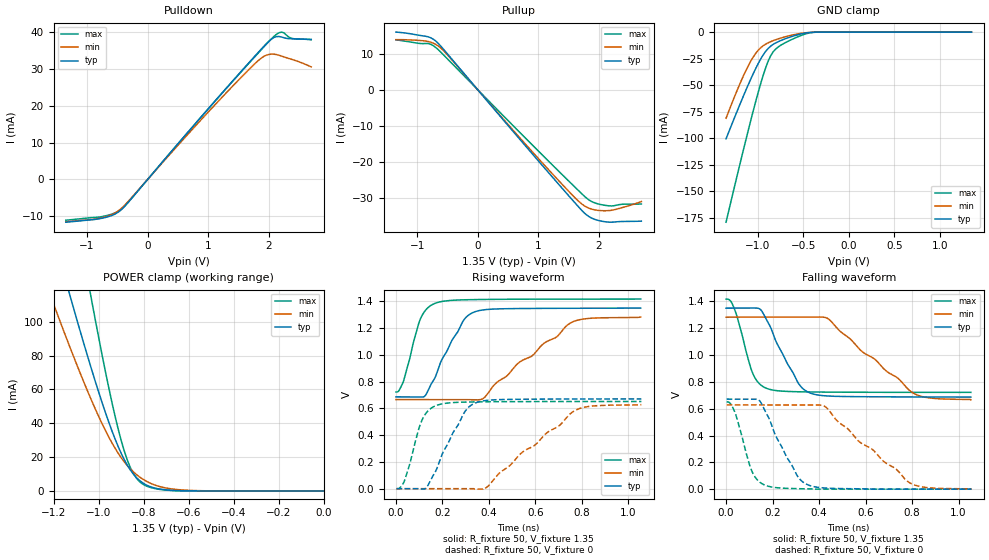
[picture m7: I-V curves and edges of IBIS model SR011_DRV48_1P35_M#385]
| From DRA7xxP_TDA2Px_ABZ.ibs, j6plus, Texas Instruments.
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| Model based on original model for DDR_SEIOPB_H
|   Sub model SR011_DRV48_1P35
[model]   SR011_DRV48_1P35_M#385
|[Description]  [1.35V-I/O-X-X]
|   , ,
|[Input Load]
|[Output Drive]
|Voltage   1.35V
|Mode   I/O
Model_type   I/O
Polarity   Non-Inverting
Enable   Active-Low
Vinl =  0.585
Vinh =  0.765
Cref =  15.0000pF
Rref =  100.0000M
Vref =  0V
Vmeas =  0.675
C_comp   2p   2p   2p
[Model Spec]
Vinl   0.585   0.55125   0.61875
Vinh   0.765   0.73125   0.79875
[Receiver Thresholds]
Tslew_ac = 5n
Vth = 0.675
Vth_max = 0.709
Vth_min = 0.608
Vinh_ac = 0.175
Vinh_dc = 0.1
Vinl_ac = -0.175
Vinl_dc = -0.1
[Temperature Range]   25   125   -40
[Voltage Range]   1.35   1.2825   1.4175
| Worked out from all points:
|   slope of the pulldown table from 0 to 0.203 V, typ, clamps not added: 51.5 ohm
|   slope of the pullup table from 0 to 0.203 V, typ, clamps not added: 50.4 ohm
|   GND clamp passes 1 mA (typ) near -0.48 V on its own axis
|   POWER clamp passes 1 mA (typ) near -0.72 V on its own axis
|   rising waveform, R_fixture 50, V_fixture 1.35: 20-80 % time 113ps typ, 274ps min, 66.1ps max; typ from 0.687 V to 1.35 V
|   rising waveform, R_fixture 50, V_fixture 0: 20-80 % time 112ps typ, 268ps min, 64.7ps max; typ from 0 V to 0.671 V
|   falling waveform, R_fixture 50, V_fixture 1.35: 20-80 % time 113ps typ, 256ps min, 66.7ps max; typ from 1.35 V to 0.687 V
|   falling waveform, R_fixture 50, V_fixture 0: 20-80 % time 113ps typ, 262ps min, 64.2ps max; typ from 0.671 V to 0 V
[POWER_clamp]
-1.35V    224.4mA    165.8mA    358.5mA
-1.214V   157mA      115.5mA    250.8mA
-1.132V   117.8mA    86.59mA    187.7mA
-1.118V   111.4mA    81.92mA    177.3mA
-1.036V   74.26mA    55.16mA    116.8mA
-954.5mV  40.7mA     31.91mA    61.06mA
-900mV    22.42mA    19.79mA    30.14mA
-859.1mV  12.48mA    13.09mA    13.96mA
-804.5mV  4.85mA     7.084mA    4.132mA
-736.4mV  1.313mA    2.9mA      1.073mA
-627.3mV  101.6uA    577.3uA    45.9uA
0V        75.63nA    322.4nA    418.5nA
[Pulldown]
-1.35V    -11.61mA   -11.5mA    -11.06mA
-736.4mV  -10.48mA   -10.33mA   -10.03mA
-531.8mV  -9.35mA    -9.062mA   -9.043mA
-409.1mV  -7.817mA   -7.49mA    -7.751mA
1.145V    21.94mA    20.88mA    21.88mA
1.718V    32.55mA    30.62mA    32.41mA
1.923V    36.25mA    33.48mA    36.08mA
2.005V    37.61mA    33.98mA    37.53mA
2.086V    38.57mA    34.03mA    38.89mA
2.209V    38.7mA     33.51mA    40.04mA
2.373V    38.22mA    32.66mA    38.36mA
2.7V      37.95mA    30.56mA    38.05mA
[Pullup]
-1.35V    15.95mA    13.86mA    13.81mA
-981.8mV  15.11mA    13.66mA    12.86mA
-818.2mV  14.65mA    13.35mA    12.79mA
-736.4mV  14.02mA    12.92mA    12.23mA
-613.6mV  12.13mA    11.6mA     10.47mA
1.064V    -20.91mA   -20.19mA   -18.01mA
1.555V    -30.35mA   -29.03mA   -26.14mA
1.759V    -34.1mA    -32.12mA   -29.45mA
1.923V    -35.82mA   -33.22mA   -31.26mA
2.168V    -36.64mA   -33.43mA   -32.13mA
2.414V    -36.45mA   -32.48mA   -31.67mA
2.7V      -36.37mA   -30.94mA   -31.63mA
[GND_clamp]
-1.35V    -100.7mA   -81.27mA   -179.3mA
-1.241V   -77.31mA   -57.61mA   -140mA
-1.132V   -54.83mA   -36.31mA   -101.6mA
-1.05V    -39.08mA   -23.36mA   -74mA
-968.2mV  -25.28mA   -14.71mA   -48.34mA
-913.6mV  -18.13mA   -11.32mA   -33.52mA
-859.1mV  -13.28mA   -9.024mA   -22.35mA
-831.8mV  -11.61mA   -8.091mA   -18.64mA
-777.3mV  -9.078mA   -6.444mA   -14.07mA
-531.8mV  -1.871mA   -1.307mA   -3.441mA
-368.2mV  -88.76uA   -111.2uA   -158uA
1.35V     75.63nA    385.5nA    349.4nA
[Ramp]
dV/dt_f 0.39858485/0.11299527n 0.37079865/0.25730624n 0.41791344/66.775518p
dV/dt_r 0.40474272/0.11278724n 0.37913037/0.27016627n 0.39238656/64.912496p
R_load = 50
[Rising Waveform]
R_fixture = 50
V_fixture = 1.35
V_fixture_min = 1.2825
V_fixture_max = 1.4175
0s        686.6mV    666.1mV    722.5mV
32.45ps   685.9mV    666mV      803.4mV
105.9ps   684.8mV    666mV      1.272V
167.7ps   828.4mV    666.1mV    1.385V
287.4ps   1.249V     665.9mV    1.412V
341.2ps   1.323V     664mV      1.414V
377.9ps   1.337V     677.4mV    1.415V
524.2ps   1.347V     936.1mV    1.416V
754.4ps   1.349V     1.242V     1.417V
1.053ns   1.35V      1.282V     1.417V
[Rising Waveform]
R_fixture = 50
V_fixture = 0
V_fixture_min = 0
V_fixture_max = 0
2.649ps   0V         0V         0V
36.95ps   0V         0V         60.29mV
113.8ps   -3.076mV   0V         518.9mV
134.2ps   15.41mV    0V         574.6mV
178.9ps   163.7mV    0V         625.4mV
294.2ps   569.7mV    0V         647.3mV
349.9ps   646.1mV    -3.001mV   649mV
391.5ps   660.3mV    11.69mV    649.8mV
773ps     670.5mV    587.2mV    651.7mV
1.055ns   671.4mV    628.3mV    651.8mV
[Falling Waveform]
R_fixture = 50
V_fixture = 1.35
V_fixture_min = 1.2825
V_fixture_max = 1.4175
0s        1.35V      1.282V     1.417V
41.14ps   1.35V      1.283V     1.321V
116.5ps   1.35V      1.283V     856.9mV
147.9ps   1.34V      1.283V     779.1mV
175ps     1.26V      1.283V     751.4mV
308.5ps   797.1mV    1.282V     726.5mV
362.2ps   716.6mV    1.283V     725mV
441ps     694.4mV    1.269V     723.7mV
808.6ps   687.7mV    713mV      722mV
1.053ns   686.6mV    666.1mV    721.8mV
[Falling Waveform]
R_fixture = 50
V_fixture = 0
V_fixture_min = 0
V_fixture_max = 0
2.649ps   671.4mV    628.3mV    650.9mV
39.77ps   671.6mV    628.3mV    565.9mV
113.6ps   671.5mV    628.4mV    124.7mV
143.6ps   660.2mV    628.4mV    54mV
170.5ps   573.2mV    628.3mV    27.67mV
304.2ps   105.4mV    628.2mV    3.736mV
355.5ps   29.7mV     628.4mV    2.316mV
429.4ps   8.083mV    611.5mV    0V
793.5ps   0V         43.77mV    0V
1.055ns   0V         0V         0V
